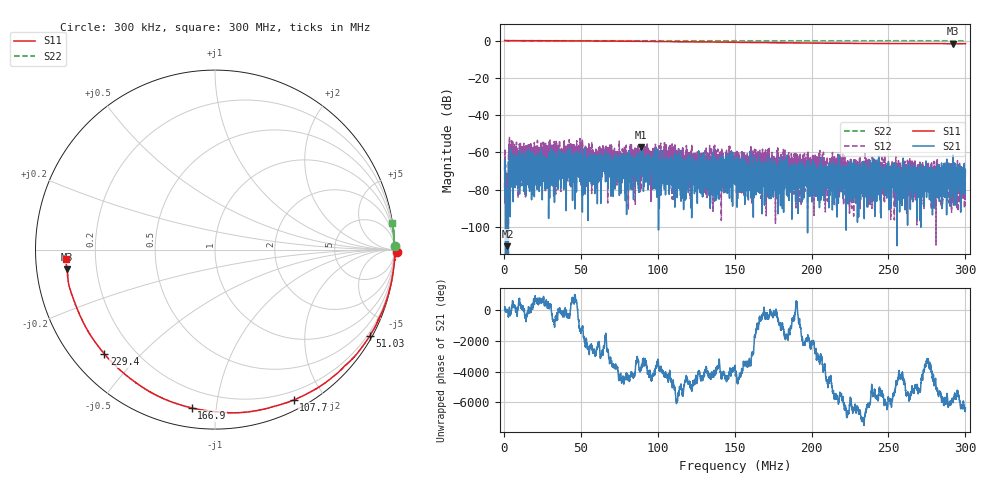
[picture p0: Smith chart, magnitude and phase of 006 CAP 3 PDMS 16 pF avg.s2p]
!  26/06/2025  15:29:40
! Ref Plane: 0.000 mm
# MHZ S MA R  50
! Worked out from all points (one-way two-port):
!   4001 points, 300 kHz to 300 MHz, reference 50 ohm
!   highest |S21| = -57.32 dB at 89.17 MHz (marker M1); lowest = -110.4 dB at 2.173 MHz (marker M2)
!   lowest |S11| = -1.6 dB at 292.1 MHz (marker M3), VSWR 10.84, Z = 4.63 - j3.31 ohm
!   |S11| at or under -10 dB: nowhere
!   |S22| runs from 0.0 to 0.1 dB; largest |S21 - S12| = 0.0031
!   S11 on the Smith chart (normalised r, x): 300 kHz: -67, -66; 51.03 MHz: 0.10, -3.85; 107.7 MHz: 0.10, -1.65; 166.9 MHz: 0.10, -0.86; 229.4 MHz: 0.10, -0.40; 300 MHz: 0.09, -0.03
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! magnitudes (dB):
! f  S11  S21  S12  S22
! 300 kHz  0.1  -69.1  -79.2  0.0
! 2.173 MHz  0.0  -110.4  -  0.0
! 4.346 MHz  0.0  -64.1  -59.1  0.0
! 8.542 MHz  0.0  -64.3  -60.2  0.0
! 12.74 MHz  0.0  -80.9  -55.2  0.0
! 16.26 MHz  0.0  -64.9  -55.0  0.0
! 50.28 MHz  -0.1  -63.2  -60.3  0.0
! 51.03 MHz  -0.1  -83.2  -56.4  0.0
! 65.11 MHz  -0.2  -63.8  -64.6  0.0
! 70.66 MHz  -0.2  -75.0  -62.9  0.0
! 89.17 MHz  -0.3  -57.3  -62.7  0.0
! 100.3 MHz  -0.4  -70.0  -73.4  0.0
! 107.7 MHz  -0.5  -68.0  -62.8  0.0
! 150.2 MHz  -0.9  -71.1  -63.2  0.0
! 166.9 MHz  -1.0  -81.2  -64.2  0.0
! 200.1 MHz  -1.3  -68.9  -63.6  0.0
! 229.4 MHz  -1.4  -71.1  -73.8  0.0
! 244.1 MHz  -1.5  -67.5  -77.0  0.0
! 250.1 MHz  -1.5  -81.6  -65.9  0.0
! 262.1 MHz  -1.6  -72.4  -70.3  0.0
! 292.1 MHz  -1.6  -75.8  -72.7  0.0
! 300 MHz  -1.6  -69.7  -76.6  0.0
